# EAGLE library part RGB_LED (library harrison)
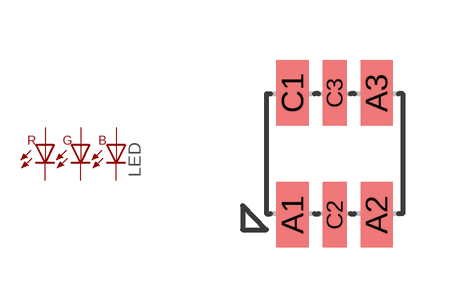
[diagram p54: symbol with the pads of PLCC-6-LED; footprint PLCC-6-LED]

Designator prefix LED

## RGB_LED_OSRAM_3MM  [PLCC-6-LED]
A1  A_R  pas
A2  A_G  pas
A3  A_B  pas
C1  C_R  pas
C2  C_G  pas
C3  C_B  pas

## Footprint PLCC-6-LED (pad centres in mm)
smd 0.8 x 1.65: A1 -1.05,-1.525; A2 1.05,-1.525; A3 1.05,1.525; C1 -1.05,1.525
smd 0.6 x 1.65: C2 0,-1.525; C3 0,1.525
